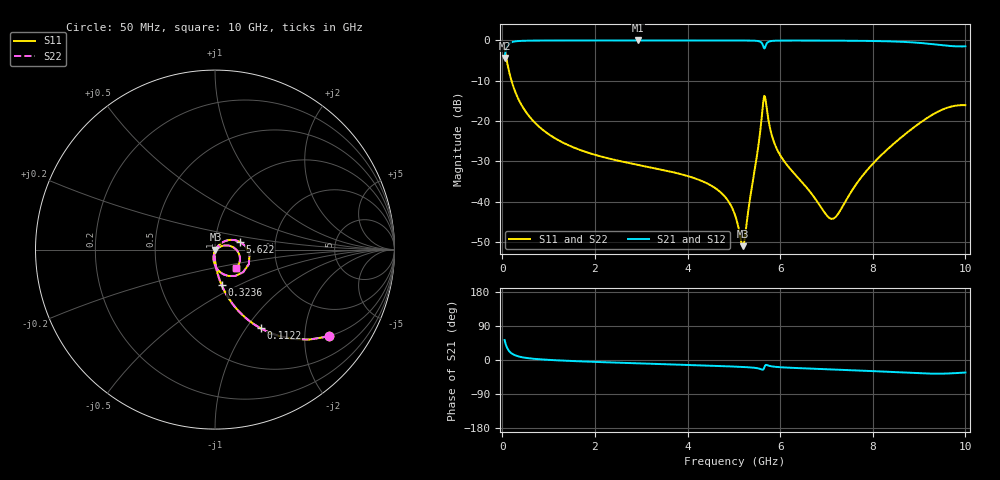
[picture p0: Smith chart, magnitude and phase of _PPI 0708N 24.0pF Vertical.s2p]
! S-Parameter data specifications (vertical orientation):
! Substrate: 40-mil Rogers 3003C, Substrate thickness, H=1.016mm, Dielectric constant, Er=3, Conductor thickness, T_mtl=0.043mm, Loss Tangent, Tand=0.003
! PCB Mounting Pad Footprint: Pad width, PadW=2.54mm , Pad length, PadL=0.51mm , Pad gap, PadG (edge-to-edge)=0.71mm , Reference planes=1.73mm apart
! Created Tue Jan 16 08:52:44 2018
# GHz S MA R 50
! 2 Port Network Data from SP1.SP block
! freq  magS11  angS11  magS21  angS21  magS12  angS12  magS22  angS22
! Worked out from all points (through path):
!   801 points, 50 MHz to 10 GHz, reference 50 ohm
!   highest |S21| = -0.01 dB at 2.923 GHz (marker M1); lowest = -4.4 dB at 50 MHz (marker M2)
!   group delay of S21, straight-line fit = 12.6 ps
!   lowest |S11| = -51.0 dB at 5.199 GHz (marker M3), VSWR 1.01, Z = 50.3 - j0.105 ohm
!   |S11| at or under -10 dB: 198.3 MHz to end of sweep
!   |S22| runs from -51.0 to -2.0 dB; largest |S21 - S12| = 0
!   S11 on the Smith chart (normalised r, x): 50 MHz: 0.99, -2.63; 112.2 MHz: 0.99, -1.17; 323.6 MHz: 0.99, -0.41; 5.622 GHz: 1.32, +0.12; 10 GHz: 1.24, -0.26
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0.05  0.797 -37.3  0.6038 52.7  0.6038 52.7  0.797 -37.3
0.1121875  0.5071 -59.9  0.8617 30.1  0.8617 30.1  0.5071 -59.9
0.1868125  0.3335 -71.2  0.9426 18.8  0.9426 18.8  0.3335 -71.2
0.323625  0.2007 -79.5  0.9794 10.4  0.9794 10.4  0.2007 -79.5
0.846  0.0802 -88.2  0.9964 1.6  0.9964 1.6  0.0802 -88.2
1.716625  0.04303 -93.1  0.9985 -3.7  0.9985 -3.7  0.04303 -93.1
2.923062  0.02865 -97.5  0.9988 -8.8  0.9988 -8.8  0.02865 -97.5
3.370812  0.02542 -98.9  0.9988 -10.6  0.9988 -10.6  0.02542 -98.9
4.539937  0.01547 -100.6  0.9984 -15.3  0.9984 -15.3  0.01547 -100.6
5.025  0.00683 -90.3  0.9978 -17.5  0.9978 -17.5  0.00683 -90.3
5.199125  0.002804 -21.9  0.997 -18.4  0.997 -18.4  0.002804 -21.9
5.497625  0.03683 48.6  0.9866 -21.4  0.9866 -21.4  0.03683 48.6
5.622  0.1451 17.5  0.8889 -25.6  0.8889 -25.6  0.1451 17.5
5.684188  0.185 -52.4  0.8492 -13.4  0.8492 -13.4  0.185 -52.4
5.821  0.06615 -95.7  0.9849 -16.8  0.9849 -16.8  0.06615 -95.7
5.995125  0.03813 -101.7  0.9942 -19.0  0.9942 -19.0  0.03813 -101.7
6.691625  0.01226 -92.9  0.9955 -22.9  0.9955 -22.9  0.01226 -92.9
7.16425  0.006234 -27.3  0.9935 -25.1  0.9935 -25.1  0.006234 -27.3
7.773688  0.0208 26.8  0.9876 -28.1  0.9876 -28.1  0.0208 26.8
8.345812  0.04614 26.2  0.9741 -31.3  0.9741 -31.3  0.04614 26.2
9.328375  0.1236 -3.0  0.8939 -36.2  0.8939 -36.2  0.1236 -3.0
10  0.1574 -41.6  0.8437 -33.1  0.8437 -33.1  0.1574 -41.6
